VAR_GLOBAL CONSTANT
	cOversamples 		: UDINT 				:= 20;								// number of oversamples
	cMaxChannels		: UDINT					:= 5;								// number of data channels
	cWindowType			: E_CM_WindowType		:= E_CM_WindowType.eCM_HannWindow;	// window type for analysis
	cWindowParameters	: T_CM_WindowParameters := [0,0,0,0,0];						// window parameters
	cWindowLength		: UDINT					:= 3200;							// length of signal window 
	cOverlap			: UDINT					:= 1600;							// recommended buffer overlap
	cBufferLength		: UDINT					:= cWindowLength - cOverlap;		// internal buffer size with 50% overlapping	                                            						
	cFFTLength			: UDINT					:= 4096;							// length of FFT for mag. spectrum
	cFFTResult			: UDINT					:= 2049;							// result of mag. spectrum (cFFTLength/2+1)
END_VAR
